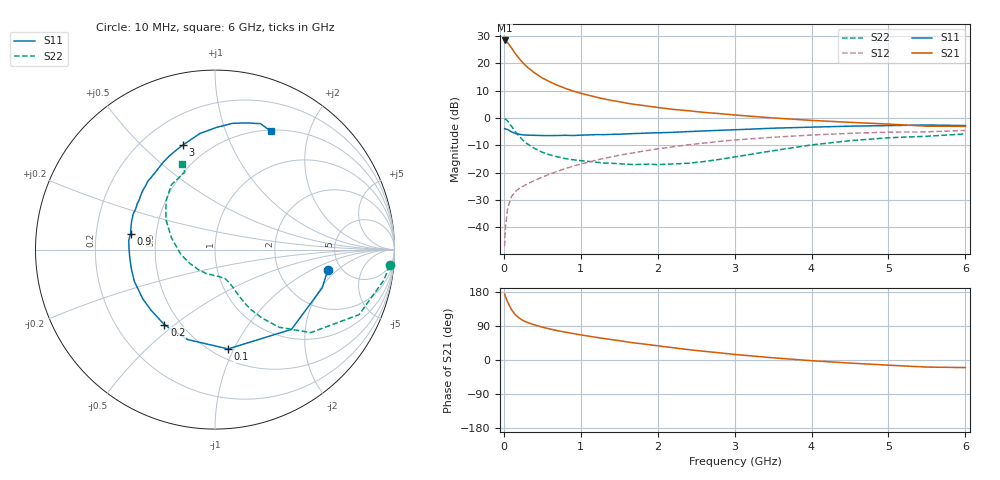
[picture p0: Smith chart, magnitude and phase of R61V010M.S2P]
! SIEMENS Small Signal Semiconductors
! BFR193
! Si NPN RF Bipolar Junction Transistor in SOT23
! VCE = 1 V  IC = 10 mA
! Common Emitter S-Parameters:  May  1996
# GHz  S  MA  R  50
!  f  S11  S21  S12  S22
! GHz  MAG  ANG  MAG  ANG  MAG  ANG  MAG  ANG
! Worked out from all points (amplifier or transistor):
!   36 points, 10 MHz to 6 GHz, reference 50 ohm
!   highest |S21| = 28.4 dB at 10 MHz (marker M1)
!   |S21| within 3 dB of that: start of sweep to 106.1 MHz
!   unconditionally stable (mu >= 1): 682.5 MHz to 2.204 GHz
!   at 250 MHz: K = 0.66, MSG = 22.6 dB, |S12| = -25.0 dB
!   at 1.4 GHz: K = 1.05, MAG = 9.0 dB, |S12| = -14.2 dB
!   at 6 GHz: K = 0.97, MSG = 0.7 dB, |S12| = -4.5 dB
!   S11 on the Smith chart (normalised r, x): 10 MHz: 3.93, -1.50; 100 MHz: 0.59, -0.95; 200 MHz: 0.41, -0.46; 900 MHz: 0.36, +0.08; 3 GHz: 0.36, +0.68; 6 GHz: 0.52, +1.45
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0.01  0.6389 -10.2  26.39 174.3  0.0045 84.9  0.9767 -5.2
0.02  0.6342 -19.6  26.05 168.2  0.0097 81.8  0.9558 -10.3
0.05  0.6157 -46.2  24.02 152.5  0.0225 70.9  0.8807 -24.3
0.1  0.5581 -82.5  19.24 132.6  0.0367 59.4  0.7062 -40.9
0.15  0.5239 -106.9  15.13 119.3  0.0451 54.1  0.5603 -50.5
0.2  0.5049 -123.9  12.29 110.7  0.0515 52.5  0.4627 -55.5
0.25  0.4909 -136.5  10.2 104.1  0.0563 52.2  0.3912 -59.0
0.3  0.487 -145.6  8.705 99.5  0.0618 53.5  0.3404 -61.0
0.4  0.4831 -158.5  6.715 92.6  0.072 55.3  0.2773 -63.1
0.5  0.4781 -167.4  5.428 86.7  0.0829 57.3  0.2368 -64.3
0.6  0.4769 -174.9  4.589 81.8  0.0945 58.7  0.2115 -65.9
0.7  0.4792 179.1  3.97 77.3  0.1062 59.7  0.1947 -67.4
0.9  0.4787 169.4  3.128 69.9  0.1314 60.0  0.1723 -70.6
1.1  0.4913 160.7  2.617 63.1  0.1559 60.0  0.1609 -76.2
1.3  0.4964 153.1  2.247 56.7  0.1823 58.8  0.1501 -82.7
1.6  0.514 143.4  1.869 47.8  0.2204 56.4  0.1426 -95.5
2.2  0.5473 126.4  1.443 32.4  0.2983 49.5  0.1445 -126.2
3  0.6102 106.9  1.138 14.7  0.3961 37.8  0.1938 -173.1
3.5  0.6522 97.4  1.005 5.8  0.4451 30.0  0.2521 164.6
4.5  0.7101 82.1  0.835 -8.1  0.5249 15.2  0.3849 135.1
5.5  0.7461 70.1  0.709 -18.7  0.5588 0.7  0.4638 111.2
6  0.7287 64.7  0.704 -20.0  0.5932 -3.6  0.5127 111.2
